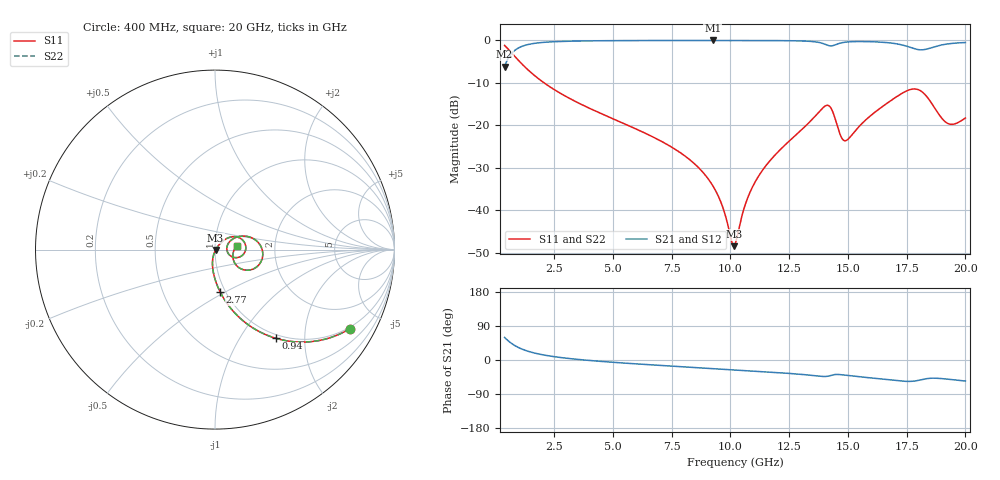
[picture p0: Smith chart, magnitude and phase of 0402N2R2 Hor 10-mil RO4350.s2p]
# MHz S  dB  R 50
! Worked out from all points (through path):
!   1961 points, 400 MHz to 20 GHz, reference 50 ohm
!   highest |S21| = -0.03 dB at 9.25 GHz (marker M1); lowest = -6.2 dB at 400 MHz (marker M2)
!   group delay of S21, straight-line fit = 11.6 ps
!   lowest |S11| = -48.4 dB at 10.15 GHz (marker M3), VSWR 1.01, Z = 50.3 - j0.179 ohm
!   |S11| at or under -10 dB: 2.08 GHz to end of sweep
!   |S22| runs from -48.4 to -1.2 dB; largest |S21 - S12| = 0
!   S11 on the Smith chart (normalised r, x): 400 MHz: 0.94, -3.44; 940 MHz: 0.94, -1.46; 2.77 GHz: 0.94, -0.47; 20 GHz: 1.27, +0.05
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400  -1.20 -30.5  -6.17 59.5  -6.17 59.5  -1.20 -30.5
940  -4.43 -55.5  -1.95 34.5  -1.95 34.5  -4.43 -55.5
1630  -8.08 -70.8  -0.74 19.0  -0.74 19.0  -8.08 -70.8
2770  -12.45 -83.0  -0.27 6.6  -0.27 6.6  -12.45 -83.0
3670  -15.09 -88.8  -0.15 0.7  -0.15 0.7  -15.09 -88.8
6940  -23.37 -101.8  -0.04 -13.9  -0.04 -13.9  -23.37 -101.8
8350  -28.41 -104.8  -0.04 -19.2  -0.04 -19.2  -28.41 -104.8
9250  -34.14 -102.8  -0.03 -22.5  -0.03 -22.5  -34.14 -102.8
9660  -38.93 -96.0  -0.04 -24.1  -0.04 -24.1  -38.93 -96.0
10150  -48.39 -27.9  -0.04 -25.9  -0.04 -25.9  -48.39 -27.9
10200  -48.05 -11.8  -0.04 -26.1  -0.04 -26.1  -48.05 -11.8
10670  -38.08 42.4  -0.04 -27.8  -0.04 -27.8  -38.08 42.4
11190  -32.04 49.1  -0.05 -29.9  -0.05 -29.9  -32.04 49.1
13470  -18.66 37.5  -0.28 -40.6  -0.28 -40.6  -18.66 37.5
14190  -15.37 -0.6  -1.25 -42.2  -1.25 -42.2  -15.37 -0.6
14710  -22.64 -13.9  -0.61 -38.7  -0.61 -38.7  -22.64 -13.9
14910  -23.59 5.6  -0.43 -40.2  -0.43 -40.2  -23.59 5.6
16740  -14.51 23.3  -0.58 -52.2  -0.58 -52.2  -14.51 23.3
17930  -11.49 -13.3  -2.12 -54.6  -2.12 -54.6  -11.49 -13.3
18420  -13.67 -33.6  -1.96 -48.7  -1.96 -48.7  -13.67 -33.6
19220  -19.45 -21.1  -0.87 -50.4  -0.87 -50.4  -19.45 -21.1
20000  -18.27 9.4  -0.53 -55.5  -0.53 -55.5  -18.27 9.4
